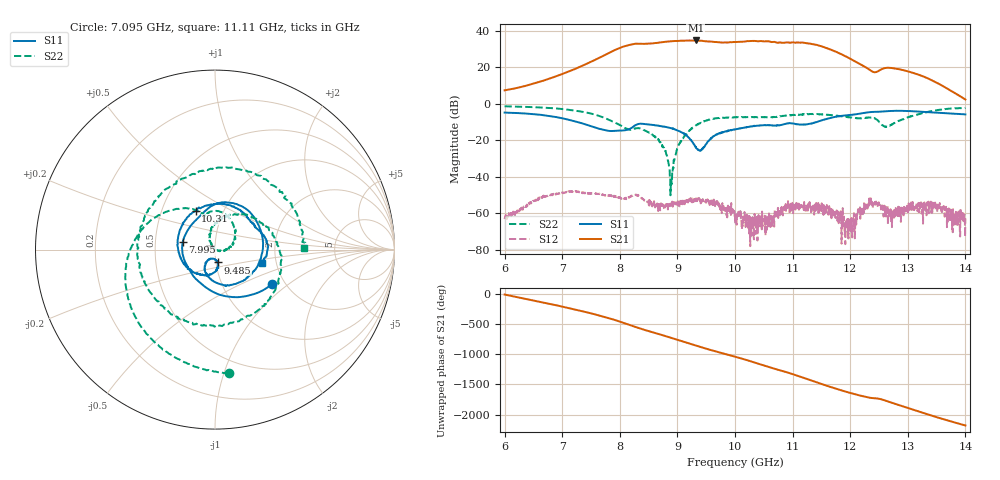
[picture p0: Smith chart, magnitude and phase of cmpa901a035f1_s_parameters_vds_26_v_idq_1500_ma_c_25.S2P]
!Keysight Technologies,E5071C,MY46110325,B.14.03
!Date: Wed Mar 10 10:59:42 2021
!Data & Calibration Information:
!Freq	S11:SOLT2(ON)	S21:SOLT2(ON)	S12:SOLT2(ON)	S22:SOLT2(ON)
!PortZ  Port1:50+j0  Port2:50+j0
!Above PortZ is port z conversion or system Z0 setting when saving the data.
!When reading, reference impedance value at option line is always used.
# Hz S dB R 50
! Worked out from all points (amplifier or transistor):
!   1601 points, 6 GHz to 14 GHz, reference 50 ohm
!   highest |S21| = 34.8 dB at 9.32 GHz (marker M1)
!   |S21| within 3 dB of that: 8.105 GHz to 11.48 GHz (3.371 GHz wide, 34.4 % of centre)
!   unconditionally stable (mu >= 1): start of sweep to end of sweep
!   at 7.33 GHz: K = 7.50, MAG = 23.0 dB, |S12| = -48.8 dB
!   at 10 GHz: K = 8.50, MAG = 34.9 dB, |S12| = -60.5 dB
!   at 14 GHz: K = 154.47, MAG = 7.7 dB, |S12| = -62.9 dB
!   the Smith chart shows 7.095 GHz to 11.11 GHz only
!   S11 on the Smith chart (normalised r, x): 7.095 GHz: 1.71, -0.77; 7.995 GHz: 0.69, +0.06; 9.485 GHz: 1.02, -0.15; 10.31 GHz: 0.74, +0.34; 11.11 GHz: 1.68, -0.27
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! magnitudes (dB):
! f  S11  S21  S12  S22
! 6 GHz  -4.8  7.4  -63.3  -1.3
! 7.095 GHz  -8.6  17.5  -48.2  -3.2
! 7.335 GHz  -10.6  20.7  -48.7  -4.3
! 7.995 GHz  -14.7  30.6  -51.3  -11.5
! 8.285 GHz  -11.5  33.0  -49.8  -13.4
! 8.67 GHz  -12.0  33.6  -54.9  -19.9
! 8.79 GHz  -12.6  34.0  -56.8  -25.9
! 8.89 GHz  -13.4  34.3  -54.1  -41.7
! 9.03 GHz  -15.0  34.6  -54.2  -22.1
! 9.32 GHz  -23.6  34.8  -52.0  -11.9
! 9.485 GHz  -22.7  34.3  -53.2  -9.4
! 10 GHz  -14.0  33.9  -60.5  -7.4
! 10.31 GHz  -12.4  34.5  -62.4  -7.3
! 11.11 GHz  -11.3  33.6  -57.3  -6.1
! 11.34 GHz  -10.8  32.8  -58.6  -5.5
! 11.61 GHz  -8.1  30.4  -58.1  -6.0
! 11.94 GHz  -6.3  25.9  -63.6  -7.2
! 12.05 GHz  -6.0  23.8  -62.6  -7.7
! 12.34 GHz  -4.5  18.6  -52.1  -7.5
! 12.67 GHz  -4.0  19.7  -61.7  -12.2
! 13.38 GHz  -4.6  13.6  -55.7  -4.3
! 14 GHz  -5.8  2.4  -62.9  -2.2
